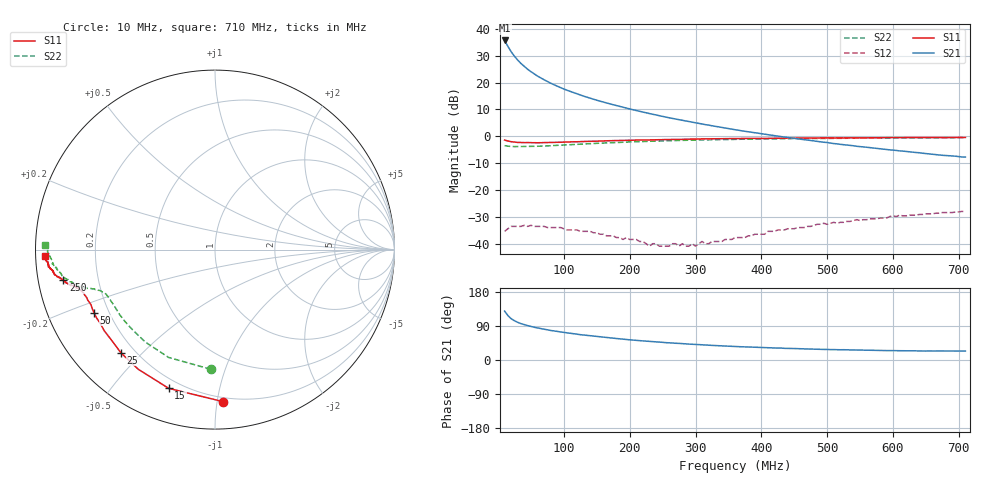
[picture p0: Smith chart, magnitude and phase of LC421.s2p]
!  POLYFET RF DEVICES
!  LC421
!  S PARAMETERS
!  VDS=12.5V, IDQ=250mA
! Date: Thu Jul 20 14:13:45 2000
! SCATTERING PARAMETERS :
# MHZ S MA R 50
!FREQ-MHZ MAG[S11] ANG[S11] MAG[S21] ANG[S21] MAG[S12] ANG[S12] MAG[S22] ANG[S22] MAG[S11] ANG[S11] MAG[S22] ANG[S22]
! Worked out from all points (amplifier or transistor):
!   141 points, 10 MHz to 710 MHz, reference 50 ohm
!   highest |S21| = 35.6 dB at 10 MHz (marker M1)
!   |S21| within 3 dB of that: start of sweep to 16.98 MHz
!   unconditionally stable (mu >= 1): 212.8 MHz to 453.4 MHz
!   at 125 MHz: K = 0.47, MSG = 25.4 dB, |S12| = -35.4 dB
!   at 360 MHz: K = 1.31, MAG = 16.7 dB, |S12| = -37.7 dB
!   at 710 MHz: K = 0.79, MSG = 10.2 dB, |S12| = -28.2 dB
!   S11 on the Smith chart (normalised r, x): 10 MHz: 0.17, -1.04; 15 MHz: 0.15, -0.71; 25 MHz: 0.15, -0.43; 50 MHz: 0.14, -0.24; 250 MHz: 0.07, -0.10; 710 MHz: 0.03, -0.02
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10  0.848 -87.0  60.6 129.1  0.017 36.6  0.667 -92.0
15  0.815 -108.5  47.02 117.2  0.019 29.7  0.654 -113.2
20  0.792 -122.7  37.32 108.9  0.021 22.6  0.645 -126.9
25  0.778 -132.4  30.75 103.6  0.021 19.1  0.641 -135.5
30  0.766 -138.9  26.05 99.3  0.021 14.1  0.642 -141.5
35  0.765 -143.8  22.49 95.9  0.021 10.3  0.643 -145.8
40  0.76 -147.4  19.85 93.2  0.022 9.5  0.642 -148.9
45  0.762 -150.3  17.63 90.8  0.021 8.1  0.643 -151.5
50  0.76 -152.5  15.9 88.5  0.022 5.5  0.646 -153.2
60  0.756 -156.0  13.17 84.6  0.021 1.9  0.651 -155.9
70  0.763 -158.4  11.25 81.3  0.021 0.8  0.656 -157.8
80  0.765 -160.1  9.701 77.9  0.02 -2.2  0.667 -159.1
95  0.773 -162.0  8.028 74.0  0.02 -3.1  0.682 -160.5
105  0.78 -162.8  7.159 71.7  0.018 -2.6  0.692 -161.2
130  0.799 -164.5  5.581 65.9  0.017 -3.5  0.719 -162.2
175  0.829 -166.0  3.857 57.4  0.014 0.7  0.761 -163.8
245  0.86 -168.4  2.409 47.3  0.009 25.0  0.814 -167.0
250  0.862 -168.6  2.334 46.6  0.009 24.9  0.819 -167.3
360  0.905 -171.4  1.323 35.8  0.013 76.0  0.875 -171.7
480  0.929 -174.0  0.816 28.6  0.022 88.5  0.906 -175.7
595  0.942 -176.0  0.558 24.9  0.032 95.8  0.929 -178.8
710  0.948 -177.8  0.409 23.6  0.039 97.0  0.946 178.5
